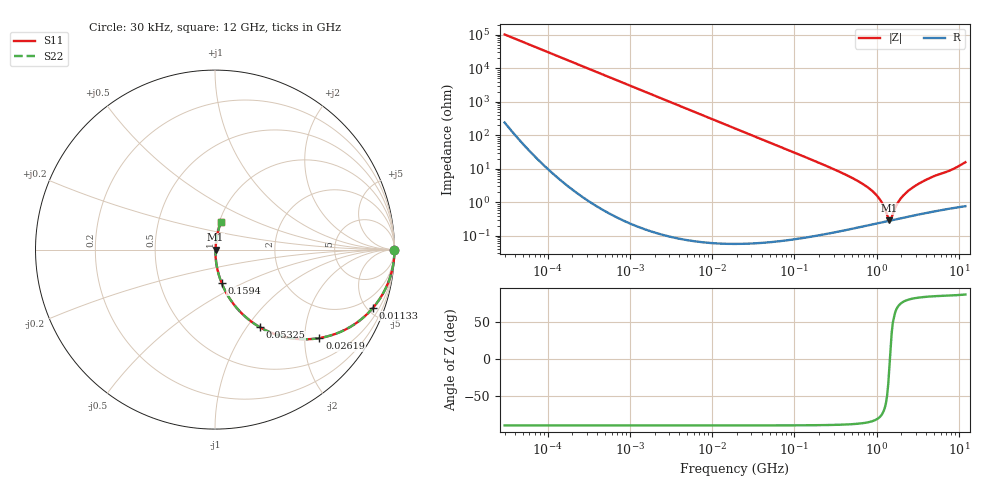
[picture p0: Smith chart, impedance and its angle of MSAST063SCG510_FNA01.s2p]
! MSAST063SCG510_FNA01  S-PARAMETER MODEL  ( Standard Model )
! Model Generated by TAIYO YUDEN Corporation (http://www.ty-top.com)
! Version 1.0
! TAIYO YUDEN Control No. 241122
! Copyright(c) 2024 TAIYO YUDEN CO.,LTD. All Rights Reserved.
! Product Description (link to TY-COMPAS)
! https://ds.yuden.co.jp/TYCOMPAS/or/detail?pn=MSAST063SCG510JFNA01&u=M
! Products Name : Multilayer Ceramic Capacitors
! Characteristics :
!  Capacitance : 51 [pF] , Rated Voltage : 25 [V] , TCC : CG / C0G
!  Case Size : 0.6 x 0.3 / 0.024 x 0.012 [mm/inch] , Thickness : 0.3 / 0.012 [mm/inch]
!  (Conditions: Temperature = 25 [degC] , DC Bias Voltage = 0 [V])
! External Node Assignments :
!  1  o---| |---o  2
! GND o---------o GND
! Frequency Range : 0.03MHz  -  12000MHz  [ 401 STEP ]
# MHZ S RI R 50
! Freq[MHz].  S11 Real  S11 Imag  S21 Real  S21 Imag  S12 Real  S12 Imag  S22 Real  S22 Imag
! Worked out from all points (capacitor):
!   401 points, 30 kHz to 12 GHz, reference 50 ohm
!   read as one part in series: C = 51.5 pF near 32 kHz
!   lowest |Z| = 290 mohm at 1.428 GHz (marker M1)
!   series resonance near 1.448 GHz, so ESL is about 230 pH
!   S11 on the Smith chart (normalised r, x): 30 kHz: open; 11.33 MHz: 1.00, -5.46; 26.19 MHz: 1.00, -2.36; 53.25 MHz: 1.00, -1.16; 159.4 MHz: 1.00, -0.38; 12 GHz: 1.02, +0.32
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0.03  1 -0.000971  3.23e-06 0.000971  3.23e-06 0.000971  1 -0.000971
0.260295  0.9999 -0.00842  7.2e-05 0.00842  7.2e-05 0.00842  0.9999 -0.00842
2.258455  0.9947 -0.0727  0.00532 0.0727  0.00532 0.0727  0.9947 -0.0727
5.223303  0.9722 -0.1643  0.0278 0.1643  0.0278 0.1643  0.9722 -0.1643
11.3258  0.8815 -0.3231  0.1185 0.3231  0.1185 0.3231  0.8815 -0.3231
18.97367  0.7261 -0.4458  0.2739 0.4458  0.2739 0.4458  0.7261 -0.4458
26.19406  0.5817 -0.493  0.4183 0.493  0.4183 0.493  0.5817 -0.493
53.24956  0.2517 -0.4334  0.7483 0.4334  0.7483 0.4334  0.2517 -0.4334
86.37604  0.1133 -0.3159  0.8867 0.3159  0.8867 0.3159  0.1133 -0.3159
159.401  0.0362 -0.1844  0.9638 0.1844  0.9638 0.1844  0.0362 -0.1844
164.6252  0.0341 -0.1788  0.9659 0.1788  0.9659 0.1788  0.0341 -0.1788
447.3588  0.0054 -0.062  0.9946 0.062  0.9946 0.062  0.0054 -0.062
799.3715  0.0028 -0.0267  0.9972 0.0267  0.9972 0.0267  0.0028 -0.0267
1103.571  0.00261 -0.0116  0.9974 0.0116  0.9974 0.0116  0.00261 -0.0116
1383.045  0.00279 -0.00191  0.9972 0.00191  0.9972 0.00191  0.00279 -0.00191
1428.372  0.00284 -0.000539  0.9972 0.000539  0.9972 0.000539  0.00284 -0.000539
1523.532  0.00294 0.00205  0.9971 -0.00205  0.9971 -0.00205  0.00294 0.00205
1733.294  0.0032 0.00739  0.9968 -0.00739  0.9968 -0.00739  0.0032 0.00739
1971.936  0.00353 0.0128  0.9965 -0.0128  0.9965 -0.0128  0.00353 0.0128
2635.962  0.00456 0.0255  0.9954 -0.0255  0.9954 -0.0255  0.00456 0.0255
4275.791  0.00753 0.0505  0.9925 -0.0505  0.9925 -0.0505  0.00753 0.0505
12000  0.0315 0.1521  0.9685 -0.1521  0.9685 -0.1521  0.0315 0.1521
